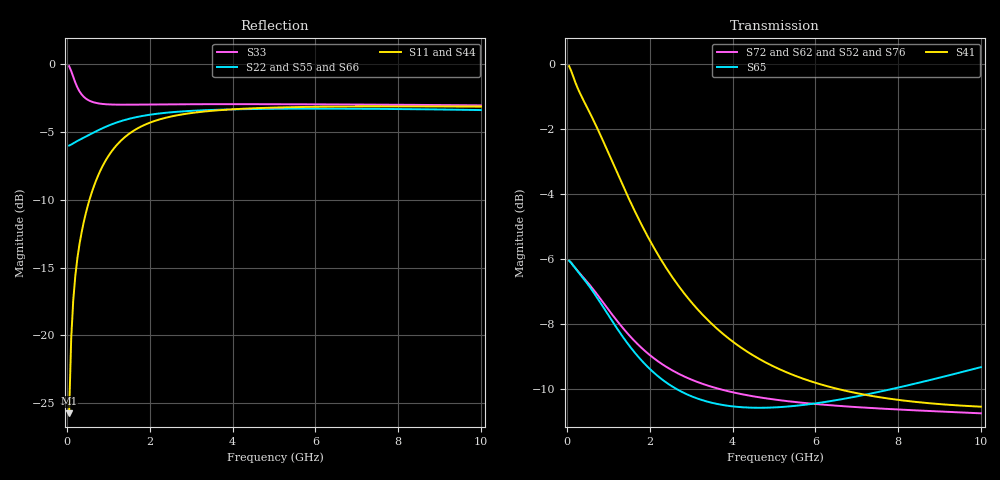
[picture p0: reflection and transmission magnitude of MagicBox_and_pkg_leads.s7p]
! Created Tue Nov 27 15:46:32 2018
# ghz S ma R 50
! 7 Port Network Data from SP1.SP block
! freq  magS11  angS11  magS12  angS12  magS13  angS13  magS14  angS14
!  magS15  angS15  magS16  angS16  magS17  angS17
!  magS21  angS21
!  magS22  angS22  magS23  angS23  magS24  angS24  magS25  angS25
!  magS26  angS26  magS27  angS27
!  magS31  angS31  magS32  angS32
!  magS33  angS33  magS34  angS34  magS35  angS35  magS36  angS36
!  magS37  angS37
!  magS41  angS41  magS42  angS42  magS43  angS43
!  magS44  angS44  magS45  angS45  magS46  angS46  magS47  angS47
!  magS51  angS51  magS52  angS52  magS53  angS53  magS54  angS54
!  magS55  angS55  magS56  angS56  magS57  angS57
!  magS61  angS61
!  magS62  angS62  magS63  angS63  magS64  angS64  magS65  angS65
!  magS66  angS66  magS67  angS67
!  magS71  angS71  magS72  angS72
!  magS73  angS73  magS74  angS74  magS75  angS75  magS76  angS76
!  magS77  angS77
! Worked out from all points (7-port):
!   200 points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, 50 MHz to 10 GHz, reference 50 ohm
!   strongest paths, dB at 50 MHz, 2.55 GHz, 5.05 GHz, 7.55 GHz, 10 GHz:
!     S41: -0.1, -6.6, -9.3, -10.2, -10.5
!     S65: -6.0, -9.9, -10.6, -10.1, -9.3
!     S72: -6.0, -9.4, -10.3, -10.6, -10.7
!     S62: -6.0, -9.4, -10.4, -10.8, -11.0
!     S52: -6.0, -9.4, -10.4, -10.8, -11.1
!     S76: -6.0, -9.7, -10.6, -10.8, -10.8
!   lowest |S11| = -25.7 dB at 50 MHz (marker M1), VSWR 1.11, Z = 49 - j5.01 ohm
!   |S11| at or under -10 dB: start of sweep to 541.8 MHz
